(* Logix 5000 AddOnInstructionDefinition export; software revision 16.04 *)

ADD_ON_INSTRUCTION AMCI_ANG1E_Absolute_Move   (* revision 1.1, vendor AMCI, ExecuteEnableInFalse *)
// Revision note:
// Version 1.1 added the slot_axis number and the input parameters can now be tags or discrete values.
VAR_INPUT
   Axis_Status_Bits : INT; {required}
   slot_axis_number : INT; {required}
   Type_0_for_standard_1_for_indexed : BOOL;
   Target_Position : DINT; {required}
   Programmed_Speed : DINT; {required}
   Acceleration : INT; {required}
   Deceleration : INT; {required}
   Jerk : INT;
END_VAR
VAR_IN_OUT
   AMCI_ANG1E_output_data : INT[10]; {required}
END_VAR
VAR_OUTPUT
   EN : BOOL; {visible}
   ER : BOOL; {visible}
END_VAR
VAR
   Upper_Result_X_1000 : DINT;
   command_data_block : INT[10];
        [0]   // Command Bits MSW
        [1]   // Command Bits LSW
        [2]   // Upper Target Position
        [3]   // Lower Target Position
        [4]   // Upper Programmed Speed
        [5]   // Lower Programmed Speed
   index : INT;
END_VAR

ROUTINE EnableInFalse   (* ladder *)
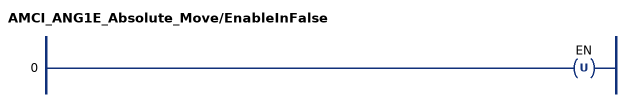
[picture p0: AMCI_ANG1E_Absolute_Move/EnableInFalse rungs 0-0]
   0: OTU(EN);
END_ROUTINE

ROUTINE Logic   (* ladder *)
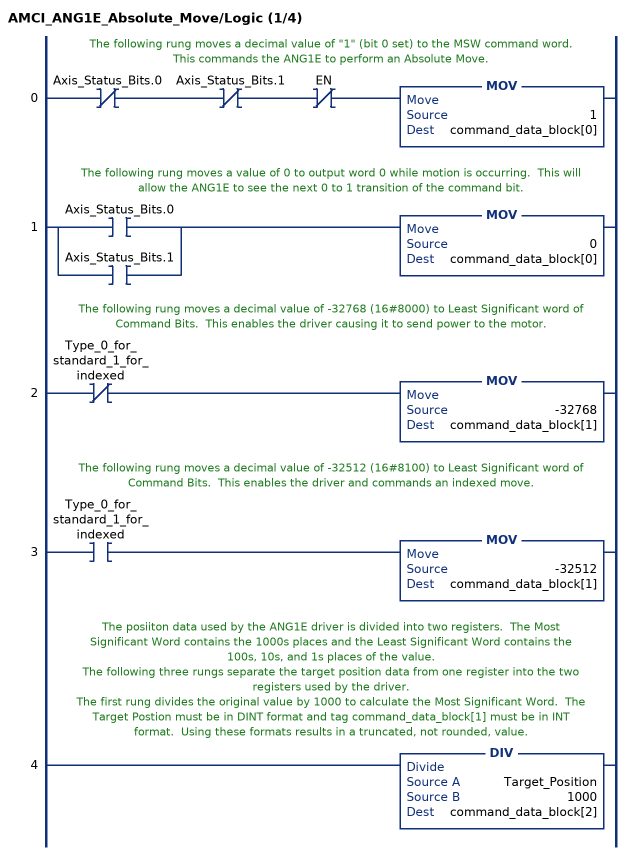
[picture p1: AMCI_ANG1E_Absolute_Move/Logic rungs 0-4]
   // The following rung moves a decimal value of "1" (bit 0 set) to the MSW command word.  This commands the ANG1E to perform an Absolute Move.
   0: XIO(Axis_Status_Bits.0)XIO(Axis_Status_Bits.1)XIO(EN)MOV(1,command_data_block[0]);
   // The following rung moves a value of 0 to output word 0 while motion is occurring.  This will allow the ANG1E to see the next 0 to 1 transition of the command bit.
   1: [XIC(Axis_Status_Bits.0) ,XIC(Axis_Status_Bits.1) ]MOV(0,command_data_block[0]);
   // The following rung moves a decimal value of -32768 (16#8000) to Least Significant word of Command Bits.  This enables the driver causing it to send power to the motor.
   2: XIO(Type_0_for_standard_1_for_indexed)MOV(-32768,command_data_block[1]);
   // The following rung moves a decimal value of -32512 (16#8100) to Least Significant word of Command Bits.  This enables the driver and commands an indexed move.
   3: XIC(Type_0_for_standard_1_for_indexed)MOV(-32512,command_data_block[1]);
   // The posiiton data used by the ANG1E driver is divided into two registers.  The Most Significant Word contains the 1000s places and the Least Significant Word contains the 100s, 10s, and 1s places of the value.
   // The following three rungs separate the target position data from one register into the two registers used by the driver.
   // The first rung divides the original value by 1000 to calculate the Most Significant Word.  The Target Postion must be in DINT format and tag command_data_block[1] must be in INT format.  Using these formats results in a truncated, not rounded, value.
   4: DIV(Target_Position,1000,command_data_block[2]);
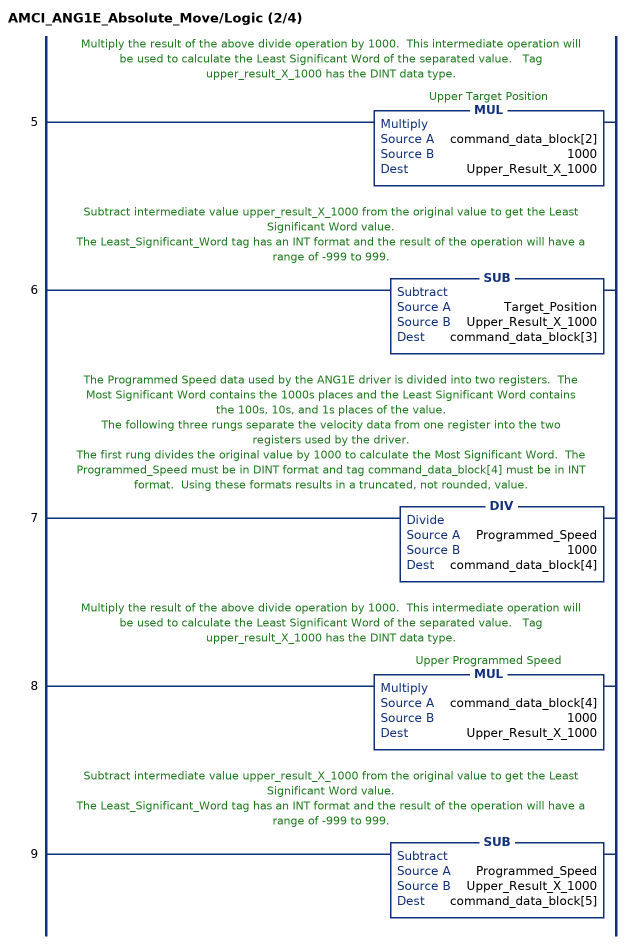
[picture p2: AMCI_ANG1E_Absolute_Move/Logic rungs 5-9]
   // Multiply the result of the above divide operation by 1000.  This intermediate operation will be used to calculate the Least Significant Word of the separated value.   Tag upper_result_X_1000 has the DINT data type.
   5: MUL(command_data_block[2],1000,Upper_Result_X_1000);
   // Subtract intermediate value upper_result_X_1000 from the original value to get the Least Significant Word value.
   // The Least_Significant_Word tag has an INT format and the result of the operation will have a range of -999 to 999.
   6: SUB(Target_Position,Upper_Result_X_1000,command_data_block[3]);
   // The Programmed Speed data used by the ANG1E driver is divided into two registers.  The Most Significant Word contains the 1000s places and the Least Significant Word contains the 100s, 10s, and 1s places of the value.
   // The following three rungs separate the velocity data from one register into the two registers used by the driver.
   // The first rung divides the original value by 1000 to calculate the Most Significant Word.  The Programmed_Speed must be in DINT format and tag command_data_block[4] must be in INT format.  Using these formats results in a truncated, not rounded, value.
   7: DIV(Programmed_Speed,1000,command_data_block[4]);
   // Multiply the result of the above divide operation by 1000.  This intermediate operation will be used to calculate the Least Significant Word of the separated value.   Tag upper_result_X_1000 has the DINT data type.
   8: MUL(command_data_block[4],1000,Upper_Result_X_1000);
   // Subtract intermediate value upper_result_X_1000 from the original value to get the Least Significant Word value.
   // The Least_Significant_Word tag has an INT format and the result of the operation will have a range of -999 to 999.
   9: SUB(Programmed_Speed,Upper_Result_X_1000,command_data_block[5]);
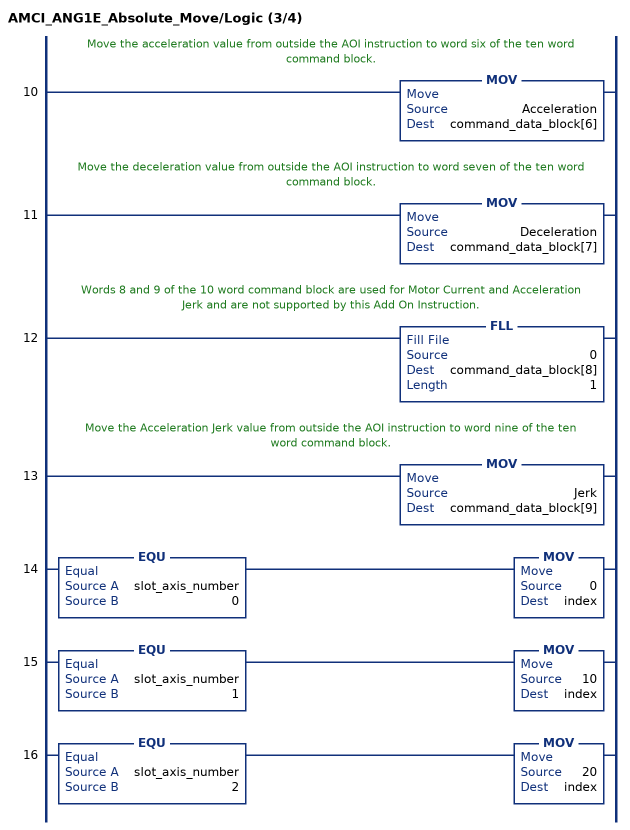
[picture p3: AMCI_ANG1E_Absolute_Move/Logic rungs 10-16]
   // Move the acceleration value from outside the AOI instruction to word six of the ten word command block.
   10: MOV(Acceleration,command_data_block[6]);
   // Move the deceleration value from outside the AOI instruction to word seven of the ten word command block.
   11: MOV(Deceleration,command_data_block[7]);
   // Words 8 and 9 of the 10 word command block are used for Motor Current and Acceleration Jerk and are not supported by this Add On Instruction.
   12: FLL(0,command_data_block[8],1);
   // Move the Acceleration Jerk value from outside the AOI instruction to word nine of the ten word command block.
   13: MOV(Jerk,command_data_block[9]);
   14: EQU(slot_axis_number,0)MOV(0,index);
   15: EQU(slot_axis_number,1)MOV(10,index);
   16: EQU(slot_axis_number,2)MOV(20,index);
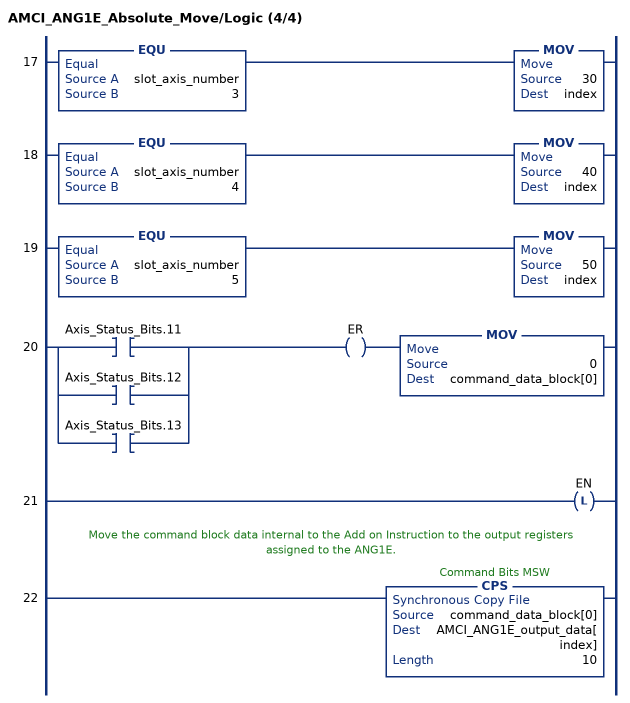
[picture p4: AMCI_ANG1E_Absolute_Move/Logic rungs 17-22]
   17: EQU(slot_axis_number,3)MOV(30,index);
   18: EQU(slot_axis_number,4)MOV(40,index);
   19: EQU(slot_axis_number,5)MOV(50,index);
   20: [XIC(Axis_Status_Bits.11) ,XIC(Axis_Status_Bits.12) ,XIC(Axis_Status_Bits.13) ]OTE(ER)MOV(0,command_data_block[0]);
   21: OTL(EN);
   // Move the command block data internal to the Add on Instruction to the output registers assigned to the ANG1E.
   22: CPS(command_data_block[0],AMCI_ANG1E_output_data[index],10);
END_ROUTINE
END_ADD_ON_INSTRUCTION
